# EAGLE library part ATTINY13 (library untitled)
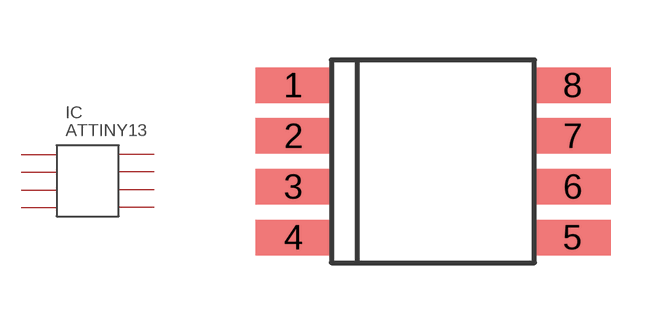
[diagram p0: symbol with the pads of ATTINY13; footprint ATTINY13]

Designator prefix IC

## ATTINY13  [ATTINY13]
1  1
2  2
3  3
4  4
5  5
6  6
7  7
8  8

## Footprint ATTINY13 (pad centres in mm)
smd 1.905 x 0.889: 1 -4.763,2.54; 2 -4.763,1.27; 3 -4.763,0; 4 -4.763,-1.27; 5 2.223,-1.27; 6 2.223,0; 7 2.223,1.27; 8 2.223,2.54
